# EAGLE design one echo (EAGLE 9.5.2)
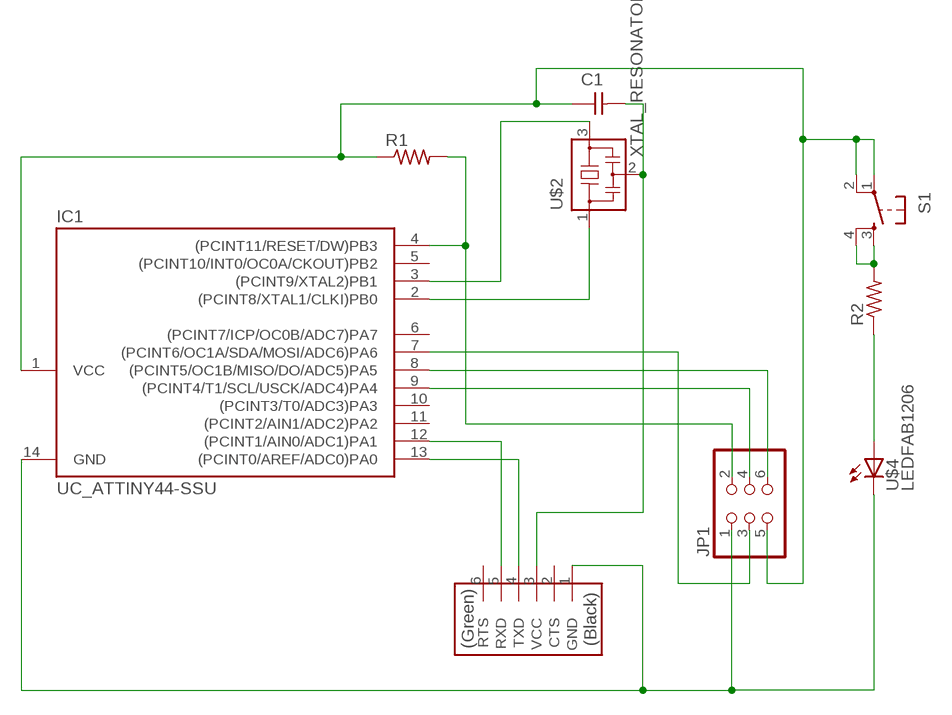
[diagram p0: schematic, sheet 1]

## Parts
C1  CAP_UNPOLARIZEDFAB  [C1206FAB]
IC1  UC_ATTINY44-SSU  [SOIC14]
JP1  CONN_03X2-PINHEAD-SMD  [2X03SMD]
R1  R1206FAB  [R1206FAB]
R2  R1206FAB  [R1206FAB]
S1  SW_SWITCH_TACTILE_6MM6MM_SWITCH  [6MM_SWITCH]
U$2  XTAL_RESONATOR  [EFOBM]
U$3  CONN_06_FTDI-SMD-HEADER  [1X06SMD]
U$4  LEDFAB1206  [LED1206FAB]

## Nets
N$1: IC1.13((PCINT0/AREF/ADC0)PA0) U$3.4(TXD)
N$2: IC1.12((PCINT1/AIN0/ADC1)PA1) U$3.5(RXD)
N$3: IC1.9((PCINT4/T1/SCL/USCK/ADC4)PA4) JP1.4
N$4: IC1.8((PCINT5/OC1B/MISO/DO/ADC5)PA5) JP1.6
N$5: IC1.14(GND) JP1.1 U$3.1(GND) U$4.2(C)
N$6: IC1.4((PCINT11/RESET/DW)PB3) JP1.2 R1.2
N$7: C1.1 IC1.1(VCC) JP1.5 R1.1 S1.1(P) S1.2(P1)
N$8: IC1.3((PCINT9/XTAL2)PB1) U$2.3
N$9: IC1.2((PCINT8/XTAL1/CLKI)PB0) U$2.1
N$10: C1.2 U$2.2 U$3.3(VCC)
N$11: IC1.7((PCINT6/OC1A/SDA/MOSI/ADC6)PA6) JP1.3
N$12: R2.1 U$4.1(A)
N$13: R2.2 S1.3(S) S1.4(S1)
Unconnected: IC1.5((PCINT10/INT0/OC0A/CKOUT)PB2) IC1.6((PCINT7/ICP/OC0B/ADC7)PA7) IC1.10((PCINT3/T0/ADC3)PA3) IC1.11((PCINT2/AIN1/ADC2)PA2) U$3.2(CTS) U$3.6(RTS)

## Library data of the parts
C1 = eagle_fab:CAP_UNPOLARIZED
IC1 = eagle_fab:UC_ATTINY44
JP1 = eagle_fab:CONN_03X2-PINHEAD-SMD: PIN HEADER
R1 R2 = eagle_fab:R: Resistor (US Symbol)
S1 = eagle_fab:SW_SWITCH_TACTILE_6MM: OMRON SWITCH
U$2 = eagle_fab:XTAL_RESONATOR
U$3 = eagle_fab:CONN_06_FTDI-SMD-HEADER
U$4 = eagle_fab:LED: LED

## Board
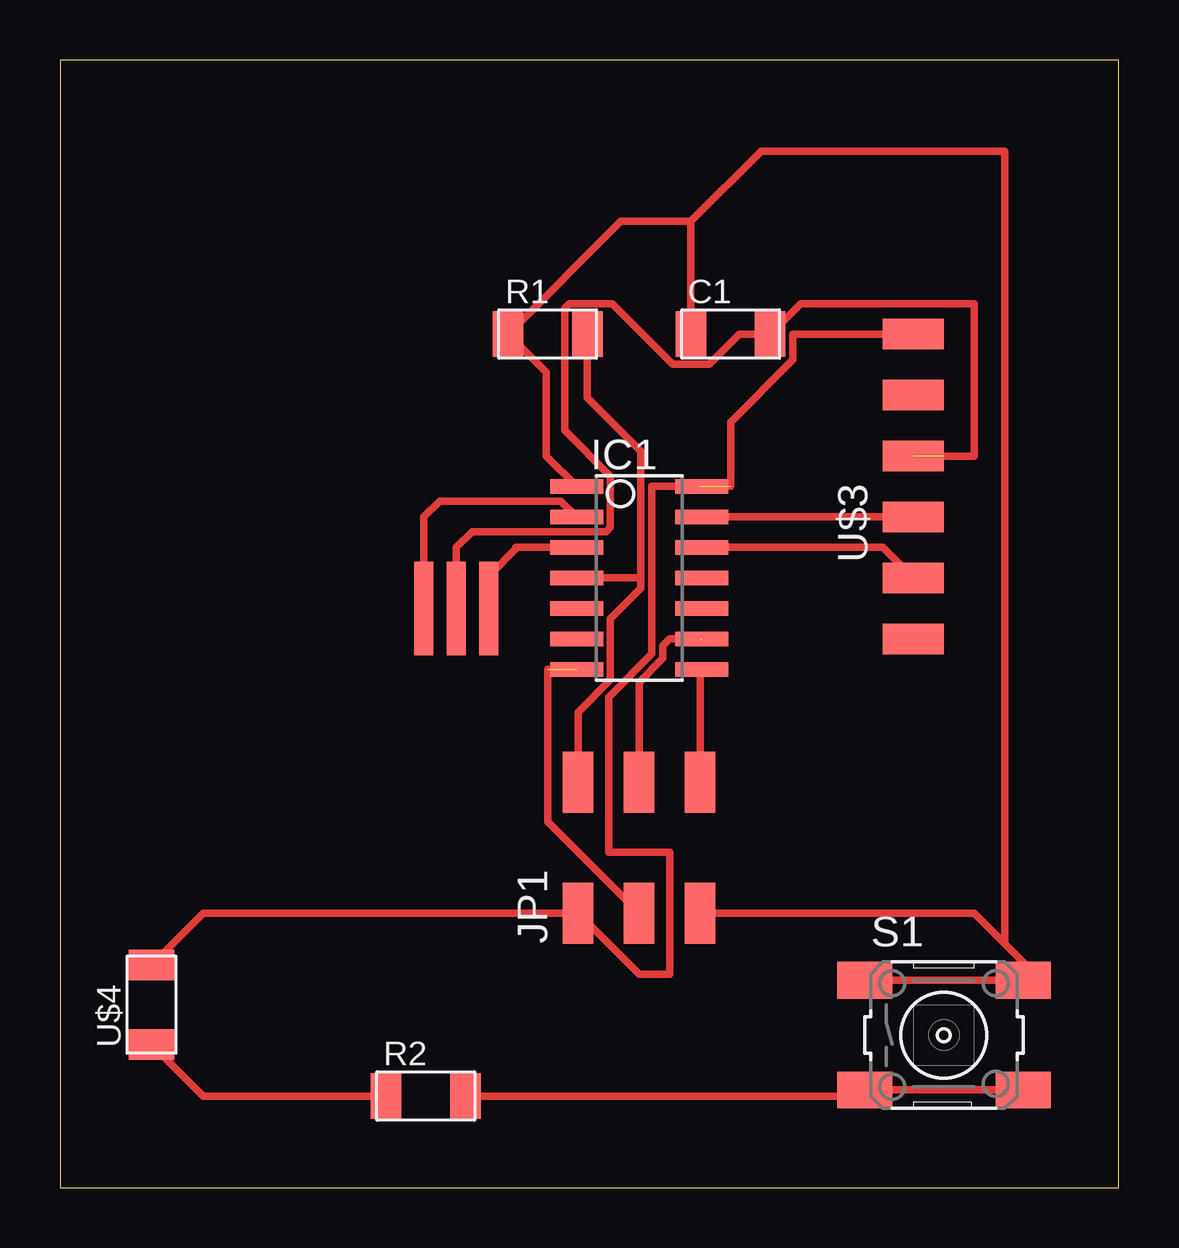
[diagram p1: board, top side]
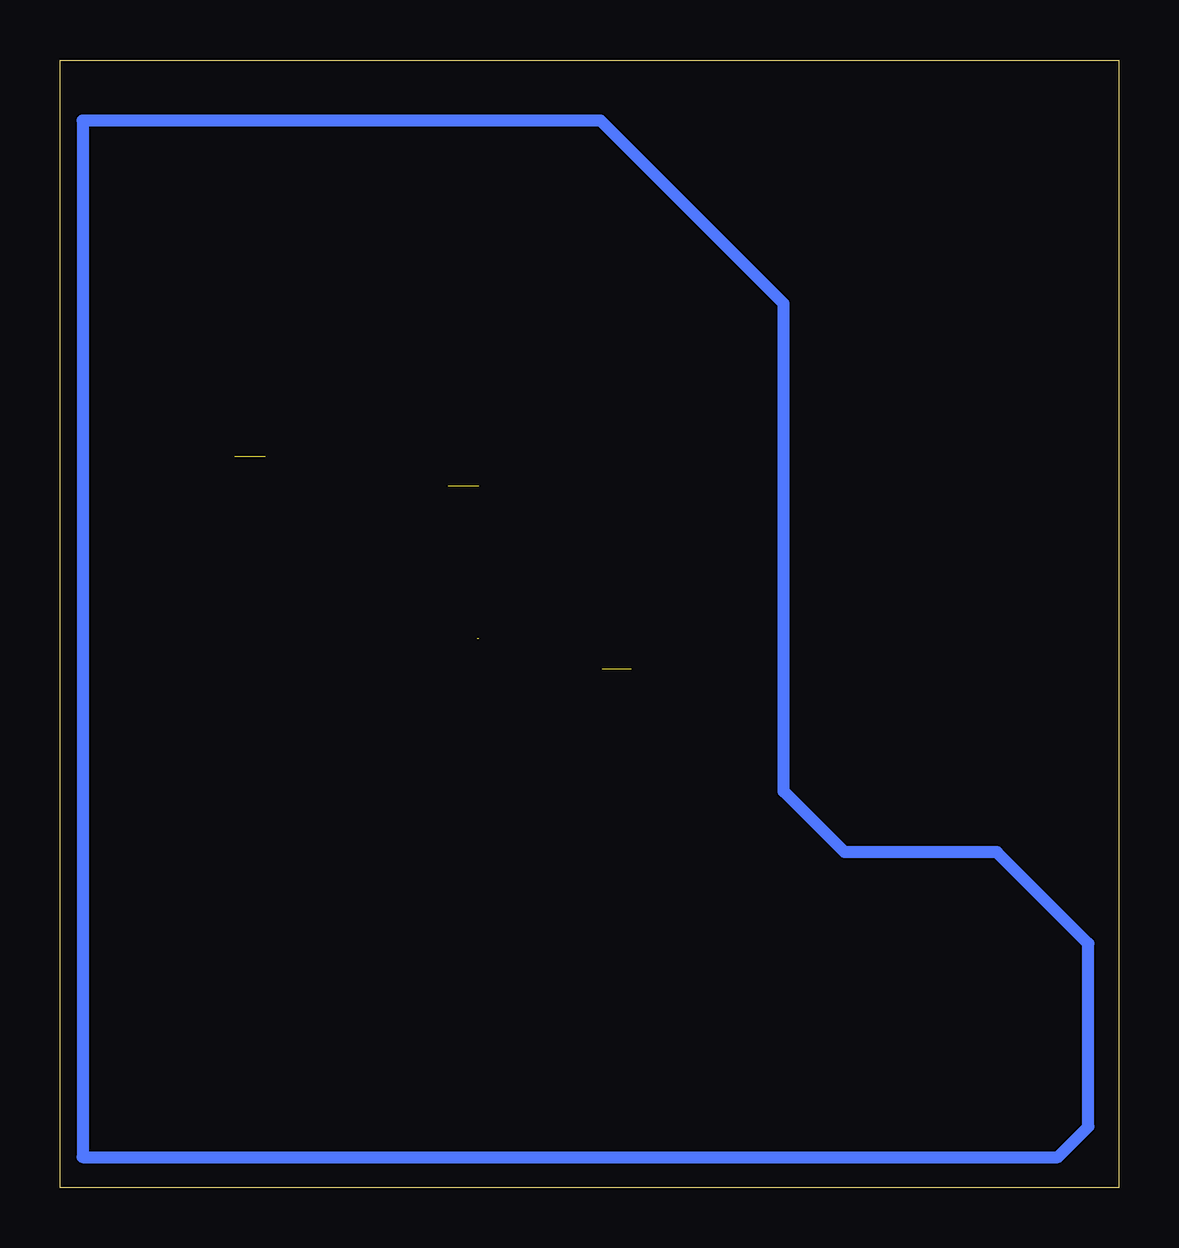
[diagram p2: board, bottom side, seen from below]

Size 44.12 x 46.98 mm. Coordinates in mm from the lower left corner, seen from the top.
Outline: 0,0 44.12,0 44.12,46.98 0,46.98 0,0
Copper layers (1*16): Top 0.035mm / dielectric 1.5mm / Bottom 0.035mm
Design rules "default": minimum track width 6mil, minimum drill 0.35mm, track to track 6mil, track to pad 6mil, pad to pad 6mil, via to via 6mil, smd to smd 6mil, copper to edge 40mil, drill to drill 6mil, minimum pad ring 10mil, minimum via ring 8mil, stop-mask expansion 4mil, vias tented up to drill 0mil, thermal gap 10mil

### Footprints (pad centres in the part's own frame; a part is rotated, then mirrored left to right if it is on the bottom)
C1206FAB = smd 1.27 x 1.905: 1 -1.651,0; 2 1.651,0
SOIC14 = smd 0.61 x 2.21: 1 -3.81,-2.603; 2 -2.54,-2.603; 3 -1.27,-2.603; 4 0,-2.603; 5 1.27,-2.603; 6 2.54,-2.603; 7 3.81,-2.603; 8 3.81,2.603; 9 2.54,2.603; 10 1.27,2.603; 11 0,2.603; 12 -1.27,2.603; 13 -2.54,2.603; 14 -3.81,2.603
2X03SMD = smd 2.54 x 1.27: 1 -2.54,2.54; 2 2.92,2.54; 3 -2.54,0; 4 2.92,0; 5 -2.54,-2.54; 6 2.92,-2.54
R1206FAB = smd 1.27 x 1.905: 1 -1.651,0; 2 1.651,0
6MM_SWITCH = smd 2.286 x 1.524: 1 -3.302,2.286; 2 3.302,2.286; 3 -3.302,-2.286; 4 3.302,-2.286
EFOBM = smd 0.8 x 3.9: 1 -1.35,0; 2 0,0; 3 1.35,0
1X06SMD = smd 2.54 x 1.27: 1 0,6.35; 2 0,3.81; 3 0,1.27; 4 0,-1.27; 5 0,-3.81; 6 0,-6.35
LED1206FAB = smd 1.27 x 1.905: 1 -1.651,0; 2 1.651,0

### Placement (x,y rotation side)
C1  27.94,35.56 0 top
IC1  24.13,25.4 270 top
JP1  24.13,13.97 90 top
R1  20.32,35.56 0 top
R2  15.24,3.81 0 top
S1  36.83,6.35 0 top
U$2  16.51,24.13 0 top
U$3  35.56,29.21 0 top
U$4  3.81,7.62 90 top

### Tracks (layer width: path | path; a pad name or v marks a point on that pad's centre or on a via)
N$1
  Top 0.305: IC1.13 U$3.4
N$2
  Top 0.305: IC1.12 34.29,26.67 U$3.5
N$3  (1 unrouted)
  Top 0.305: 26.67,22.86 25.4,22.86 25.12,22.58 25.12,22.05 24.13,21.06 JP1.4
N$4
  Top 0.305: JP1.6 26.67,21.53 IC1.8
N$5  (2 unrouted)
  Top 0.305: U$3.1 30.53,35.56 30.53,34.48 27.94,31.89 27.94,29.21 | U$4.2 5.97,11.43 JP1.1 24.13,8.89 25.4,8.89 25.4,13.97 22.86,13.97 22.86,20.44 24.66,22.24 24.66,29.21 26.67,29.21
N$6
  Top 0.305: R1.2 21.97,32.91 24.21,30.67 24.21,25.4 | 24.21,25.4 24.21,24.97 22.94,23.7 22.94,21.16 21.59,19.81 JP1.2 | 24.21,25.4 IC1.4
N$7
  Top 0.305: 39.37,10.16 38.1,11.43 JP1.5 | S1.2 S1.1 40.39,8.64 40.64,8.89 39.37,10.16 | IC1.1 20.26,30.48 20.26,33.97 R1.1 23.37,40.26 26.29,40.26 | 39.37,10.16 39.37,43.18 29.21,43.18 26.29,40.26 | 26.29,40.26 C1.1
N$8
  Top 0.305: 17.86,24.27 U$2.3 17.86,25.48 19.05,26.67 | 18.99,26.67 19.05,26.67 | 19.05,26.67 IC1.3
N$9
  Top 0.305: IC1.2 20.87,28.6 15.82,28.6 15.16,27.94 U$2.1
N$10  (1 unrouted)
  Top 0.305: 36.83,30.48 38.1,30.48 38.1,36.83 30.86,36.83 C1.2 28.31,35.56 27.05,34.3 25.53,34.3 23.01,36.82 21.21,36.82 21.03,36.64 21.03,31.55 22.94,29.64 22.94,27.51 22.76,27.33 17.17,27.33 16.51,26.67 U$2.2
N$11  (1 unrouted)
  Top 0.305: JP1.3 20.32,15.24 20.32,21.59
N$12
  Top 0.305: U$4.1 5.97,3.81 R2.1
N$13
  Top 0.305: S1.4 S1.3 33.27,3.81 R2.2
N$14
  Bottom 0.508: 1.27,2.54 1.27,10.16 5.08,13.97 11.43,13.97 13.97,16.51 13.97,36.83 21.59,44.45 43.18,44.45 43.18,1.27 2.54,1.27 1.27,2.54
